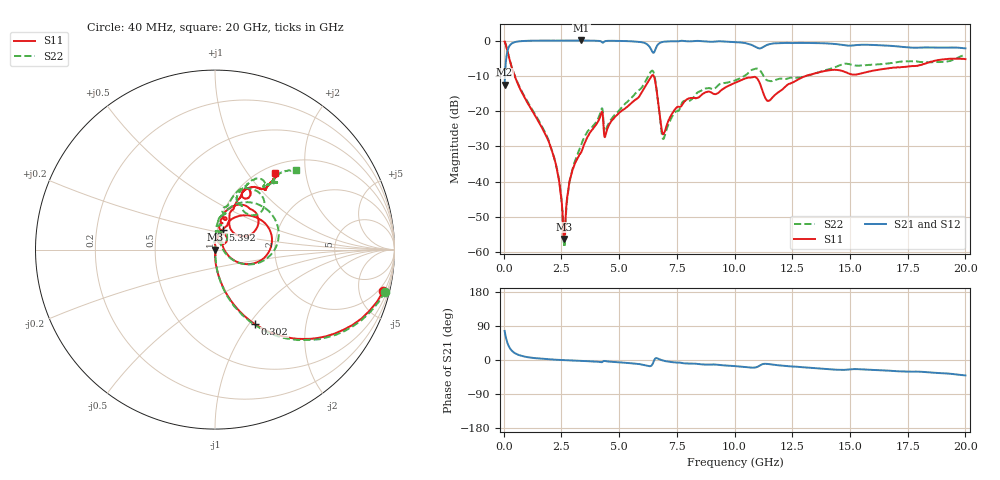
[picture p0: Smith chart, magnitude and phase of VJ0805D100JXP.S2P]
! VJ0805D100JXP
! DATE 10/29/2021  12:00
! CAPACITORS MOUNTED IN SERIES ON 25 MIL THICK MICROSTRIP SUBSTRATE
# GHz  S  MA  R  50.00
!  FREQ  S11M  S11A  S21M  S21A  S12M  S12A  S22M  S22A
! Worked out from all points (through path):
!   1601 points, 40 MHz to 20 GHz, reference 50 ohm
!   highest |S21| = 0.03 dB at 3.358 GHz (marker M1); lowest = -12.5 dB at 40 MHz (marker M2)
!   group delay of S21, straight-line fit = 6.51 ps
!   lowest |S11| = -56.2 dB at 2.61 GHz (marker M3), VSWR 1.00, Z = 50.2 - j0.0386 ohm
!   |S11| at or under -10 dB: 472.8 MHz to 6.408 GHz (5.935 GHz wide, 173 % of centre); 6.496 GHz to 13.09 GHz (6.592 GHz wide, 67.3 % of centre)
!   |S22| runs from -58.2 to -0.2 dB; largest |S21 - S12| = 0.0072
!   S11 on the Smith chart (normalised r, x): 40 MHz: 1.16, -8.12; 302 MHz: 1.00, -1.07; 5.392 GHz: 1.06, +0.24; 20 GHz: 1.13, +1.37
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0.04  0.9665 -13.8  0.2363 76.7  0.2374 76.4  0.9757 -13.9
0.301975  0.4706 -61.8  0.881 28.2  0.8812 28.1  0.4762 -62.0
0.71365  0.2064 -78.4  0.9787 11.9  0.9788 11.9  0.2113 -78.7
2.036  0.03109 -84.8  0.9973 1.5  0.9977 1.4  0.0308 -87.8
2.3853  0.01085 -83.0  0.9972 0.3  0.9977 0.3  0.0113 -84.3
2.60985  0.001552 -14.3  0.9974 -0.3  0.9984 -0.4  0.001231 -41.7
2.921725  0.0124 79.2  0.9983 -1.1  0.9991 -1.2  0.0126 91.4
3.35835  0.02616 88.0  1.003 -2.2  1.004 -2.4  0.03318 98.9
3.370825  0.02679 88.3  1.003 -2.3  1.003 -2.4  0.03416 99.5
4.194175  0.08621 72.7  0.9792 -5.6  0.9804 -5.7  0.09669 77.9
4.443675  0.05017 73.1  0.9866 -3.4  0.9865 -3.5  0.05605 77.4
5.391775  0.1187 69.0  0.9805 -7.9  0.981 -8.0  0.139 85.2
6.414725  0.3184 25.6  0.7179 -13.9  0.7184 -14.0  0.373 30.2
6.70165  0.1255 -29.6  0.8924 3.2  0.8933 3.1  0.1237 -30.1
6.938675  0.04822 30.0  0.9618 -2.1  0.9631 -2.2  0.04118 32.8
7.79945  0.1327 79.4  0.9878 -8.7  0.9878 -8.7  0.139 78.4
10.02  0.251 69.1  0.9527 -16.1  0.9525 -16.3  0.2721 73.1
10.90573  0.3036 39.6  0.8155 -19.7  0.8162 -20.0  0.3982 56.0
11.47958  0.1398 46.9  0.8824 -10.7  0.8833 -10.9  0.2688 47.9
13.35083  0.3334 64.0  0.9227 -20.8  0.9228 -21.0  0.3313 67.6
16.68165  0.4053 59.0  0.8438 -28.3  0.8442 -28.7  0.4742 50.3
20  0.5453 51.9  0.7744 -40.7  0.7743 -41.1  0.6327 44.3
